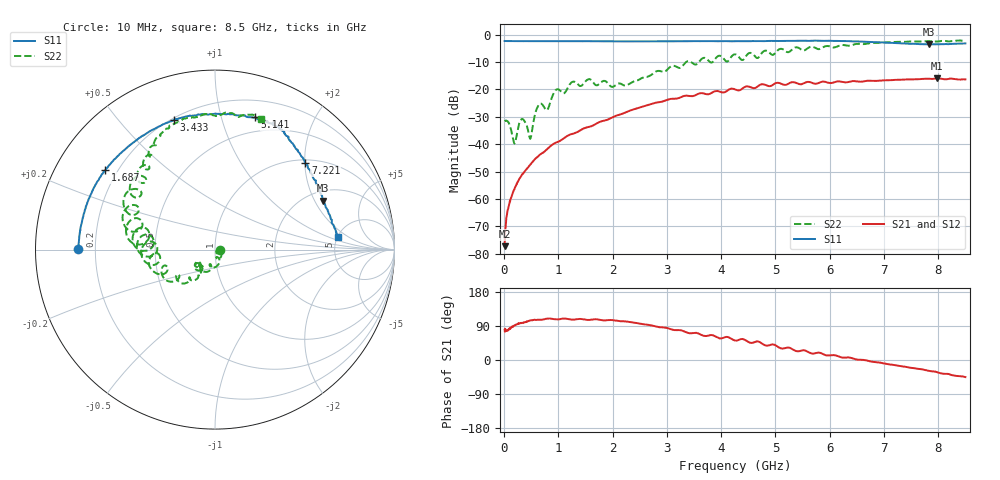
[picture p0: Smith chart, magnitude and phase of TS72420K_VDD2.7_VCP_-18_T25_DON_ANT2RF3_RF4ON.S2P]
!Agilent Technologies,E5071C,MY46417908,A.11.23
!Date: Thu Oct 03 16:41:48 2019
!Data & Calibration Information:
!Freq	S11:SOLT2(ON)	S21:SOLT2(ON)	S12:SOLT2(ON)	S22:SOLT2(ON)
!PortZ  Port1:50+j0  Port2:50+j0
!Above PortZ is port z conversion or system Z0 setting when saving the data.
!When reading, reference impedance value at option line is always used.
# Hz S dB R 50
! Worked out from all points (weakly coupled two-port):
!   1601 points, 10 MHz to 8.5 GHz, reference 50 ohm
!   highest |S21| = -15.97 dB at 7.98 GHz (marker M1); lowest = -77.2 dB at 10 MHz (marker M2)
!   lowest |S11| = -3.6 dB at 7.826 GHz (marker M3), VSWR 4.88, Z = 121 + j117 ohm
!   |S11| at or under -10 dB: nowhere
!   |S22| runs from -39.7 to -2.2 dB; largest |S21 - S12| = 0.0019
!   S11 on the Smith chart (normalised r, x): 10 MHz: 0.13, +0.00; 1.687 GHz: 0.15, +0.32; 3.433 GHz: 0.21, +0.71; 5.141 GHz: 0.36, +1.28; 7.221 GHz: 1.08, +2.02; 8.5 GHz: 5.07, +1.37
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1e7  -2.35 179.8  -77.19 79.8  -78.61 90.8  -31.60 -2.0
7.3675e7  -2.37 178.2  -63.71 77.8  -63.94 78.0  -31.79 -26.5
1.904125e8  -2.40 175.3  -56.47 91.0  -56.37 91.4  -39.74 -24.0
3.28375e8  -2.39 172.3  -51.13 97.8  -51.26 97.4  -30.76 -26.9
4.822562e8  -2.41 168.9  -47.47 104.5  -47.44 104.4  -38.03 -39.4
6.4675e8  -2.41 165.2  -44.05 106.3  -44.02 106.3  -25.44 -54.3
7.900188e8  -2.42 162.0  -41.89 109.2  -41.88 108.9  -27.59 -76.8
9.598188e8  -2.40 158.3  -39.36 107.2  -39.35 107.2  -20.11 -90.8
1.426769e9  -2.44 149.1  -34.68 108.1  -34.67 108.1  -18.67 -125.7
1.686775e9  -2.45 144.0  -32.64 107.6  -32.65 107.6  -18.41 -141.6
2.254544e9  -2.49 132.3  -28.28 101.6  -28.27 101.7  -18.53 -129.4
2.843538e9  -2.48 119.8  -24.70 86.9  -24.69 86.9  -13.25 -129.7
3.432531e9  -2.41 107.7  -22.45 70.5  -22.43 70.6  -9.88 -158.7
4.255e9  -2.43 91.5  -20.00 51.5  -19.98 51.3  -7.23 176.2
4.732562e9  -2.37 82.0  -18.19 45.3  -18.16 45.2  -7.17 176.2
5.141144e9  -2.28 73.3  -18.22 30.3  -18.15 30.2  -5.39 153.2
5.671769e9  -2.27 65.6  -17.59 17.2  -17.55 17.6  -4.43 139.1
7.088538e9  -2.99 46.5  -16.69 -11.3  -16.64 -11.0  -2.79 111.7
7.221194e9  -3.14 43.6  -16.52 -14.2  -16.51 -13.8  -2.66 110.0
7.826106e9  -3.61 24.4  -16.12 -28.6  -16.18 -28.4  -2.43 93.6
7.979988e9  -3.55 19.0  -15.97 -32.3  -16.02 -32.1  -2.56 88.4
8.5e9  -3.22 5.9  -16.35 -45.1  -16.39 -45.3  -2.23 70.6
